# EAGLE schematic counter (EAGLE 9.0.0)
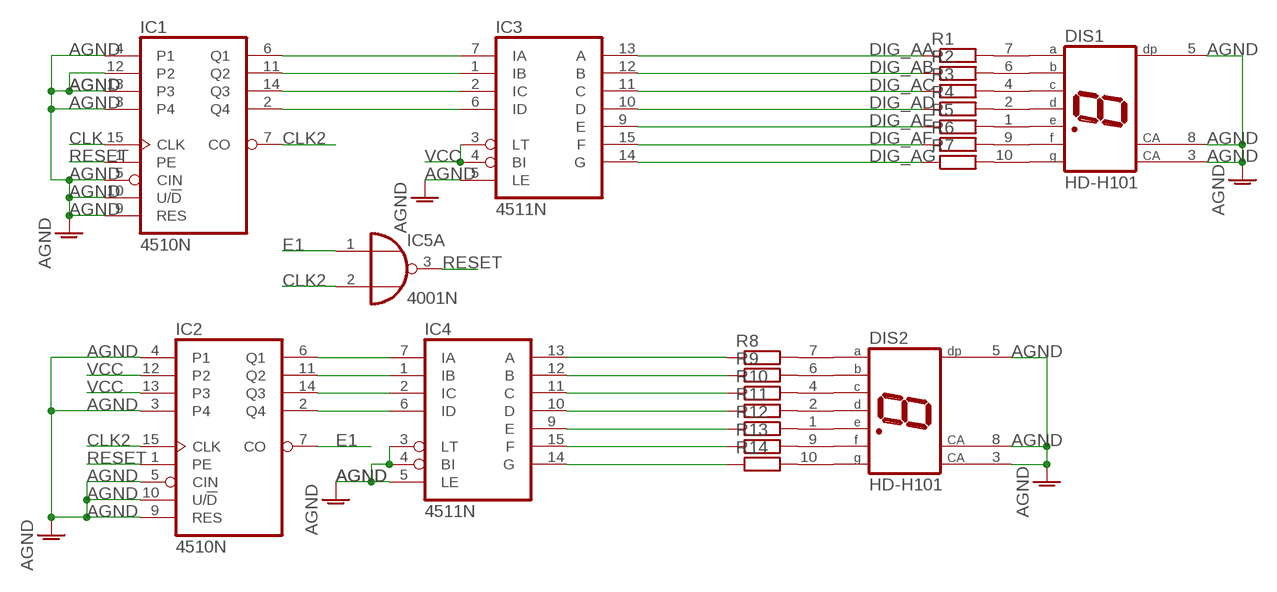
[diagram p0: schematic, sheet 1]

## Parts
DIS1  HD-H101  [HDSP-M]
DIS2  HD-H101  [HDSP-M]
IC1  4510N  [DIL16]
IC2  4510N  [DIL16]
IC3  4511N  [DIL16]
IC4  4511N  [DIL16]
IC5  4001N  [DIL14]
R1  R-EU_0207/12  [0207/12]
R2  R-EU_0207/12  [0207/12]
R3  R-EU_0207/12  [0207/12]
R4  R-EU_0207/12  [0207/12]
R5  R-EU_0207/12  [0207/12]
R6  R-EU_0207/12  [0207/12]
R7  R-EU_0207/12  [0207/12]
R8  R-EU_0207/12  [0207/12]
R9  R-EU_0207/12  [0207/12]
R10  R-EU_0207/12  [0207/12]
R11  R-EU_0207/12  [0207/12]
R12  R-EU_0207/12  [0207/12]
R13  R-EU_0207/12  [0207/12]
R14  R-EU_0207/12  [0207/12]

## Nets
AGND: DIS1.3(CA) DIS1.5(DP) DIS1.8(CA) DIS2.3(CA) DIS2.5(DP) DIS2.8(CA) IC1.3(P4) IC1.4(P1) IC1.5(CIN) IC1.9(RES) IC1.10(U/!D) IC1.12(P2) IC1.13(P3) IC2.3(P4) IC2.4(P1) IC2.5(CIN) IC2.9(RES) IC2.10(U/!D) IC3.5(LE) IC4.3(LT) IC4.4(BI) IC4.5(LE)
CLK: IC1.15(CLK)
CLK2: IC1.7(CO) IC2.15(CLK) IC5.2(A:I1)
DIG_AA: IC3.13(A) R1.1
DIG_AB: IC3.12(B) R2.1
DIG_AC: IC3.11(C) R3.1
DIG_AD: IC3.10(D) R4.1
DIG_AE: IC3.9(E) R5.1
DIG_AF: IC3.15(F) R6.1
DIG_AG: IC3.14(G) R7.1
E1: IC2.7(CO) IC5.1(A:I0)
N$2: IC1.6(Q1) IC3.7(IA)
N$3: IC1.11(Q2) IC3.1(IB)
N$4: IC1.14(Q3) IC3.2(IC)
N$5: IC1.2(Q4) IC3.6(ID)
N$6: DIS1.7(A) R1.2
N$7: DIS1.6(B) R2.2
N$8: DIS1.4(C) R3.2
N$9: DIS1.2(D) R4.2
N$10: DIS1.1(E) R5.2
N$11: DIS1.9(F) R6.2
N$12: DIS1.10(G) R7.2
N$13: DIS2.7(A) R8.2
N$14: DIS2.6(B) R9.2
N$15: DIS2.4(C) R10.2
N$16: DIS2.2(D) R11.2
N$17: DIS2.1(E) R12.2
N$18: DIS2.9(F) R13.2
N$19: DIS2.10(G) R14.2
N$20: IC2.6(Q1) IC4.7(IA)
N$21: IC2.11(Q2) IC4.1(IB)
N$22: IC2.14(Q3) IC4.2(IC)
N$23: IC2.2(Q4) IC4.6(ID)
N$24: IC4.13(A) R8.1
N$25: IC4.12(B) R9.1
N$26: IC4.11(C) R10.1
N$27: IC4.10(D) R11.1
N$28: IC4.9(E) R12.1
N$29: IC4.15(F) R13.1
N$30: IC4.14(G) R14.1
RESET: IC1.1(PE) IC2.1(PE) IC5.3(A:O)
VCC: IC2.12(P2) IC2.13(P3) IC3.3(LT) IC3.4(BI)
Unconnected: IC5.4(B:O) IC5.5(B:I0) IC5.6(B:I1) IC5.8(C:I0) IC5.9(C:I1) IC5.10(C:O) IC5.11(D:O) IC5.12(D:I0) IC5.13(D:I1)

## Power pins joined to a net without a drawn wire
VDD: IC1.16(VDD) IC2.16(VDD) IC3.16(VDD) IC4.16(VDD) IC5.14(P:VDD)
VSS: IC1.8(VSS) IC2.8(VSS) IC3.8(VSS) IC4.8(VSS) IC5.7(P:VSS)

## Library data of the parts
DIS1 DIS2 = display-hp:HD-H101: LED DISPLAY 1-character 7 segment, decimal point right; OC_FARNELL: unknown; OC_NEWARK: unknown
IC1 IC2 = 45xx:4510: BCD up down COUNTER
IC3 IC4 = 45xx:4511: BCD to 7-segment LATCH/DECODER/DRIVER
IC5 = 40xx:4001: Quad 2-input NOR
R1-R14 = resistor:R-EU_: RESISTOR, European symbol

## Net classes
0 default: clearance 0.205 mm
